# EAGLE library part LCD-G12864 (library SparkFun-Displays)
Graphical LCD 128x64 Graphical LCD 644x128 with LED Backlight. STN Type. KS0108B parallel interface chipset. Datasheet SparkFun Products: Graphic LCD 128x64
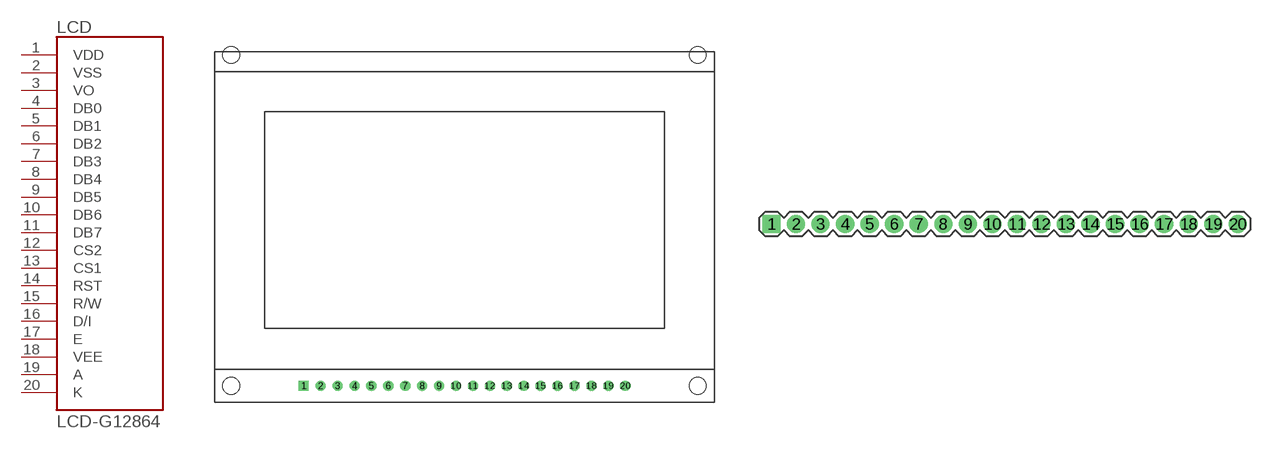
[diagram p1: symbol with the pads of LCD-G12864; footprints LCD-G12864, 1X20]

Designator prefix LCD

## LCD-G12864-FULL (SF_ID: LCD-00710)  [LCD-G12864]
1  VDD  pwr
2  VSS  pwr
3  VO
4  DB0
5  DB1
6  DB2
7  DB3
8  DB4
9  DB5
10  DB6
11  DB7
12  CS2  in
13  CS1  in
14  RST  in
15  R/W  in
16  D/I  in
17  E  in
18  VEE
19  A  pwr
20  K  pwr

## LCD-G12864-BARE (SF_ID: LCD-00710)  [1X20]
Pads as for LCD-G12864

## Footprint LCD-G12864 (pad centres in mm)
G12864 For 128x64 LCDs. Specifications: Pin count: 16 Pin pitch: 0.1" Area: Datasheet referenced for footprint: Example device(s): Basic 16x2 LCD
drill 1.016 square: 1 13.4,2.5
drill 1.016: 2 15.94,2.5; 3 18.48,2.5; 4 21.02,2.5; 5 23.56,2.5; 6 26.1,2.5; 7 28.64,2.5; 8 31.18,2.5; 9 33.72,2.5; 10 36.26,2.5; 11 38.8,2.5; 12 41.34,2.5; 13 43.88,2.5; 14 46.42,2.5; 15 48.96,2.5; 16 51.5,2.5; 17 54.04,2.5; 18 56.58,2.5; 19 59.12,2.5; 20 61.66,2.5
hole 2.5 at 2.5,2.5
hole 2.5 at 2.5,52.2
hole 2.5 at 72.5,52.2
hole 2.5 at 72.5,2.5

## Footprint 1X20 (pad centres in mm)
0.1" SIL LCD connection Specifications: Pin count: 20 Pin pitch: 0.1in Area: 0.1 x 2.0 in Example Device(s): none
drill 1.016 pad 1.88 square: 1 0,0
drill 1.016 pad 1.88: 2 2.54,0; 3 5.08,0; 4 7.62,0; 5 10.16,0; 6 12.7,0; 7 15.24,0; 8 17.78,0; 9 20.32,0; 10 22.86,0; 11 25.4,0; 12 27.94,0; 13 30.48,0; 14 33.02,0; 15 35.56,0; 16 38.1,0; 17 40.64,0; 18 43.18,0; 19 45.72,0; 20 48.26,0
